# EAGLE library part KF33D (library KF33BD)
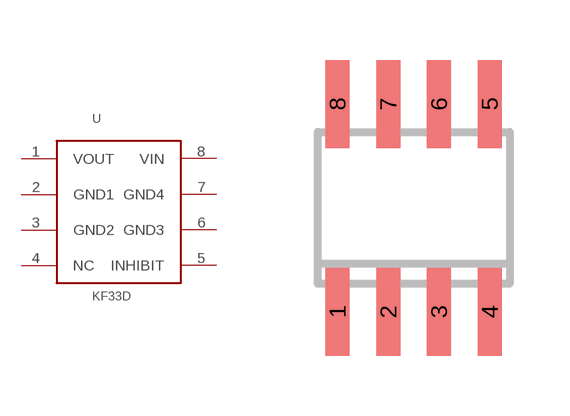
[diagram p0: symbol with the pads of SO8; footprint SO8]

Designator prefix -

## KF33D  [SO8]
1  VOUT  out
2  GND1  pwr
3  GND2  pwr
4  NC  nc
5  INHIBIT  in
6  GND3  pwr
7  GND4  pwr
8  VIN  in

## Footprint SO8 (pad centres in mm)
8-Lead Small Outline IC (SO-8) Source: http://www.analog.com/UploadedFiles/Data_Sheets/703465986AD8611_2_0.pdf
smd 0.6 x 2.2: 1 -1.905,-2.6; 2 -0.635,-2.6; 3 0.635,-2.6; 4 1.905,-2.6; 5 1.905,2.6; 6 0.635,2.6; 7 -0.635,2.6; 8 -1.905,2.6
